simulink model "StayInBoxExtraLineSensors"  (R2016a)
settings: Solver=FixedStepAuto  StartTime=0.0  StopTime=inf  RelTol=1e-3
libraries: miniQ x2

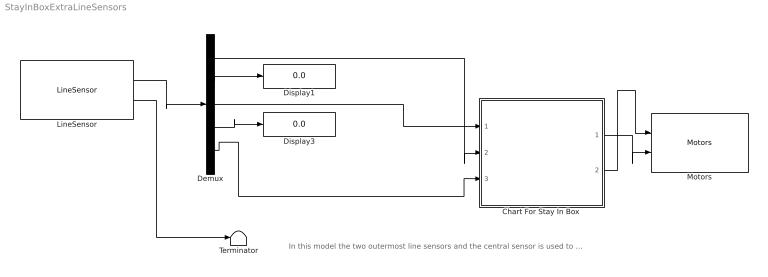
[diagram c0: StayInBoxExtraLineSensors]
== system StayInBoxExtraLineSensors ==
  note: In this model the two outermost line sensors and the central sensor is used to keep the miniQ robot within a box
  "Chart For Stay In Box " : Stateflow chart  TreatAsAtomicUnit=on
  Demux : Demux  Outputs=5
  Display1 : Display
  Display3 : Display
  LineSensor : miniQ/LineSensor  sampleTime_dd=0.01  maxRawSensors=[800,900,900,900,800]  minRawSensors=[200,280,300,300,220]  debug_dd=off
  Motors : miniQ/Motors  flipLeft=off  flipRight=off
  Terminator : Terminator
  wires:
  LineSensor/2 -> Terminator/1
  Demux/1 -> "Chart For Stay In Box "/2(SL)
  LineSensor/1 -> Demux/1
  Demux/4 -> Display3/1
  Demux/2 -> Display1/1
  Demux/5 -> "Chart For Stay In Box "/3(SR)
  Demux/3 -> "Chart For Stay In Box "/1(value)
  "Chart For Stay In Box "/1(r) -> Motors/2
  "Chart For Stay In Box "/2(l) -> Motors/1

== stateflow chart StayInBoxExtraLineSensors/Chart For Stay In Box
 ==
  state A back up and left tur is caused when the central sensor [group]
    detects a black line at the value <300
  state LeftSensor
    entry: l=-255
    r=255
  state Left
    entry: l=-150
    r=150
  state Forward
    entry: l=255
    r=255
  state Here the outermost sensors, when they hit a black line [group]
    at <500 causes a left or right turn
  state RightSensor
    entry: l=255
    r=-255
  state Backward
    entry: l=-150
    r=-150
  (default) -> Forward
  LeftSensor -> Forward : [SL>500]
  Forward -> LeftSensor : [SL<500]
  Left -> Forward : after(.5,sec)
  RightSensor -> Forward : [SR>500]
  Backward -> Left : after(.5,sec)
  Forward -> Backward : [value<300]
  Forward -> RightSensor : [SR<500]
  data: value input; r output; l output; SL input; SR input
